DATA_BLOCK     DRIVDB90
TITLE=         DRIVDB90
AUTHOR:        DRVDPS7
FAMILY:        DRIVES
NAME:          DRIVDB90
VERSION:       5.5

STRUCT
   SLAVE_3                     : STRUCT
       DPADDR                  : WORD;           // PROFIBUS address / device number of the slave
       DADDR                   : WORD;           // Diagnostics address of the slave
       SLOT_4                  : SLOT_UDT;       // Slot-specific configuration data Slot 4
       SLOT_5                  : SLOT_UDT;       // Slot-specific configuration data Slot 5
   END_STRUCT;

END_STRUCT;


BEGIN
   // SLAVE_3
   SLAVE_3.DPADDR              := W#16#3;        // PROFIBUS address / device number of the slave: 3
   SLAVE_3.DADDR               := W#16#7FE;      // Diagnostics address of the slave: 2046
   SLAVE_3.SLOT_4.LADDR        := W#16#100;      // I/O base address of the slot: 256
   SLAVE_3.SLOT_4.SLOT_ID      := B#16#2;        // Slot type designation: 2
   SLAVE_3.SLOT_4.PCD_ADDR     := B#16#1;        // Process data start address for setpoint and/or actual value slot: 1
   SLAVE_3.SLOT_4.LENGTH       := B#16#6;        // Length in words of slot data to be transferred: 6
   SLAVE_3.SLOT_4.CONSIST      := TRUE;          // Consistency: Total length
   SLAVE_3.SLOT_5.LADDR        := W#16#100;      // I/O base address of the slot: 256
   SLAVE_3.SLOT_5.SLOT_ID      := B#16#1;        // Slot type designation: 1
   SLAVE_3.SLOT_5.PCD_ADDR     := B#16#1;        // Process data start address for setpoint and/or actual value slot: 1
   SLAVE_3.SLOT_5.LENGTH       := B#16#6;        // Length in words of slot data to be transferred: 6
   SLAVE_3.SLOT_5.CONSIST      := TRUE;          // Consistency: Total length

END_DATA_BLOCK
